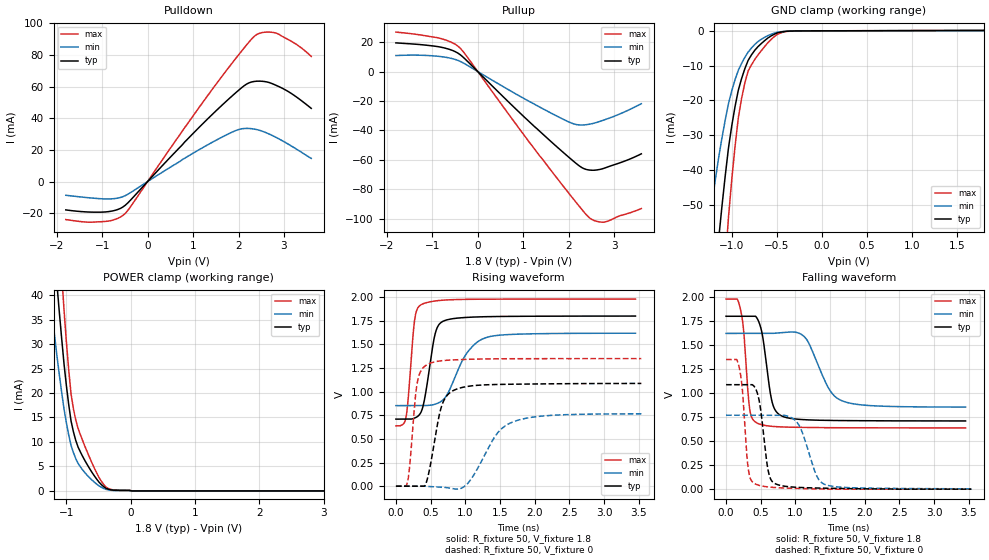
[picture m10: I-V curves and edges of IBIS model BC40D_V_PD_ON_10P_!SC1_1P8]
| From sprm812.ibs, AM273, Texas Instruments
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|   Model Cell BC40D_V_PD_ON_10P_!SC1_1P8
|BC40D_V_PD_ON_10P_!SC1_1P8
[Model]   BC40D_V_PD_ON_10P_!SC1_1P8
Model_type   I/O
Polarity   Non-Inverting
Enable   Active-Low
Vinl =  0.63
Vinh =  1.17
Cref =  15pF
Rref =  100.0000M
Vref =  0V
Vmeas =  0.9
C_comp   2.290246p   2.205796p   2.292736p
|[Input load] weak_pd_on
|[Output drive] fast
|[supplytol] 10
|[temp] ind
[Model Spec]
Vinl   0.63   0.567   0.693
Vinh   1.17   1.053   1.287
[Temperature Range]   25   125   -40
[Voltage Range]   1.8   1.62   1.98
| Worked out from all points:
|   slope of the pulldown table from 0 to 0.27 V, typ, clamps not added: 32.2 ohm
|   slope of the pullup table from 0 to 0.27 V, typ, clamps not added: 32.5 ohm
|   GND clamp passes 1 mA (typ) near -0.53 V on its own axis
|   POWER clamp passes 1 mA (typ) near -0.43 V on its own axis
|   rising waveform, R_fixture 50, V_fixture 1.8: 20-80 % time 141ps typ, 321ps min, 87.4ps max; typ from 0.709 V to 1.8 V
|   rising waveform, R_fixture 50, V_fixture 0: 20-80 % time 174ps typ, 379ps min, 98.8ps max; typ from 0 V to 1.09 V
|   falling waveform, R_fixture 50, V_fixture 1.8: 20-80 % time 128ps typ, 291ps min, 84ps max; typ from 1.8 V to 0.709 V
|   falling waveform, R_fixture 50, V_fixture 0: 20-80 % time 111ps typ, 211ps min, 81ps max; typ from 1.09 V to 0 V
| Nom Voltages:
|   VDD=1.1001, VDDS=1.8, VDDS18=1.8, ESD_BIASFET=0, VSS=0, VSSS=0
| Min Voltages:
|   VDD=0.99, VDDS=1.62, VDDS18=1.62, ESD_BIASFET=0, VSS=0, VSSS=0
| Max Voltages:
|   VDD=1.21, VDDS=1.98, VDDS18=1.98, ESD_BIASFET=0, VSS=0, VSSS=0
[POWER_clamp]
|   voltage   I(typ)   I(min)   I(max)
-1.8V     158.9mA    112.6mA    219.9mA
-1.255V   60.04mA    40.04mA    85.04mA
-1.145V   41.99mA    27.45mA    59.9mA
-1.109V   36.4mA     23.66mA    51.96mA
-1.073V   31.03mA    20.08mA    44.3mA
-1.036V   25.91mA    16.71mA    36.9mA
-927.3mV  14.27mA    9.297mA    19.77mA
-854.5mV  10.33mA    6.619mA    14.49mA
-454.5mV  1.273mA    741.7uA    1.94mA
-309.1mV  221.6uA    132.8uA    307.9uA
18.18mV   0A         0A         0A
3.6V      0A         0A         0A
[Pulldown]
|   voltage   I(typ)   I(min)   I(max)
-1.8V     -17.92mA   -8.674mA   -24.03mA
-927.3mV  -19.22mA   -10.99mA   -25.2mA
-654.5mV  -17.65mA   -10.46mA   -23.22mA
-490.9mV  -14.97mA   -8.904mA   -20.12mA
818.2mV   25.05mA    14.78mA    34.16mA
1.691V    49.7mA     28.87mA    68.58mA
2.127V    60.63mA    33.53mA    84.59mA
2.4V      63.43mA    32.85mA    92.9mA
2.618V    62.99mA    30.74mA    94.47mA
2.836V    60.69mA    27.76mA    93.76mA
3.273V    53.49mA    20.53mA    86.73mA
3.6V      46.26mA    14.64mA    79.12mA
[Pullup]
|   voltage   I(typ)   I(min)   I(max)
-1.8V     19.47mA    10.86mA    26.81mA
-818.2mV  16.61mA    10.18mA    22.5mA
-545.5mV  14.2mA     8.665mA    19.39mA
-381.8mV  11.35mA    6.855mA    15.77mA
1.036V    -31.31mA   -18.66mA   -43.94mA
1.909V    -55.72mA   -32.86mA   -78.99mA
2.182V    -62.87mA   -36.1mA    -89.59mA
2.345V    -66.12mA   -36.26mA   -95.76mA
2.455V    -66.95mA   -35.82mA   -99.33mA
2.618V    -66.9mA    -34.58mA   -101.8mA
2.782V    -65.72mA   -32.89mA   -102.4mA
3.6V      -55.92mA   -21.86mA   -93.15mA
[GND_clamp]
|   voltage   I(typ)   I(min)   I(max)
-1.8V     -270.2mA   -170.2mA   -430.1mA
-1.255V   -91.66mA   -55.91mA   -148.4mA
-1.145V   -59.91mA   -36.45mA   -97.1mA
-1.109V   -50.48mA   -30.83mA   -81.56mA
-1.073V   -41.73mA   -25.65mA   -67.06mA
-1.036V   -33.67mA   -20.93mA   -53.6mA
-927.3mV  -17.08mA   -11.35mA   -25.06mA
-854.5mV  -10.88mA   -7.623mA   -14.95mA
-781.8mV  -6.944mA   -4.955mA   -9.81mA
-636.4mV  -2.852mA   -1.883mA   -4.568mA
-381.8mV  -107.5uA   -91.83uA   -158.4uA
1.8V      101.9uA    59.86uA    152.6uA
[Ramp]
| variable   typ   min   max
dV/dt_f 0.66510519/0.13032151n 0.47058165/0.29690499n 0.81401058/85.695381p
dV/dt_r 0.66379761/0.17655114n 0.48092033/0.39577716n 0.81801831/99.528337p
R_load = 50
[Rising Waveform]
R_fixture = 50
V_fixture = 1.8
V_fixture_min = 1.62
V_fixture_max = 1.98
|   time   V(typ)   V(min)   V(max)
0s        708.5mV    851.3mV    637.8mV
143.7ps   708.5mV    851.3mV    722.4mV
176.4ps   708.5mV    851.3mV    920mV
269.4ps   719.8mV    851.3mV    1.753V
369.4ps   794.8mV    851.3mV    1.92V
561.6ps   1.599V     865.5mV    1.957V
684.8ps   1.745V     916mV      1.966V
1.012ns   1.783V     1.395V     1.974V
1.287ns   1.791V     1.567V     1.976V
3.453ns   1.798V     1.617V     1.977V
[Rising Waveform]
R_fixture = 50
V_fixture = 0
V_fixture_min = 0
V_fixture_max = 0
|   time   V(typ)   V(min)   V(max)
0s        0V         0V         0V
165.8ps   0V         0V         40.15mV
306.2ps   0V         0V         1.087V
458.3ps   91.27mV    -2.724mV   1.288V
653.5ps   834.6mV    -10.24mV   1.325V
852.6ps   1.019V     -30.77mV   1.335V
1.044ns   1.056V     37.26mV    1.341V
1.449ns   1.075V     546.9mV    1.346V
1.676ns   1.077V     676mV      1.347V
3.538ns   1.086V     764.7mV    1.348V
[Falling Waveform]
R_fixture = 50
V_fixture = 1.8
V_fixture_min = 1.62
V_fixture_max = 1.98
|   time   V(typ)   V(min)   V(max)
0s        1.798V     1.62V      1.977V
200.1ps   1.798V     1.62V      1.895V
252.3ps   1.798V     1.62V      1.658V
340.4ps   1.798V     1.62V      835.7mV
443.5ps   1.781V     1.62V      689.1mV
663.1ps   908.8mV    1.62V      653.2mV
797.3ps   763mV      1.628V     647.2mV
1.144ns   721.8mV    1.574V     642.3mV
1.673ns   713.2mV    918.6mV    638.4mV
3.453ns   709.3mV    853.4mV    637.1mV
[Falling Waveform]
R_fixture = 50
V_fixture = 0
V_fixture_min = 0
V_fixture_max = 0
|   time   V(typ)   V(min)   V(max)
0s        1.086V     769.1mV    1.348V
185.3ps   1.086V     769.1mV    1.28V
233.6ps   1.086V     769.1mV    1.048V
319.1ps   1.086V     769.1mV    218.1mV
422.3ps   1.05V      769.1mV    54.69mV
608.2ps   189.3mV    769.1mV    22.92mV
712ps     55.7mV     769.1mV    16.43mV
1.033ns   18.86mV    686.4mV    7.342mV
1.431ns   9.918mV    47.16mV    0V
3.538ns   0V         3.297mV    0V
